|Texas Instruments Incorporated
|tmux4051, 1 Data Lane 8:1 24V Precision mux
[IBIS Ver]   4.1
[File name]   tmux4051.ibs
[Date]   05/26/22
[File Rev]   1.0
[Source]
| Texas Instruments Incorporated.
| ASC-INT-MPD
| 12500 TI Blvd
| Dallas, TX - 75243
[Notes]   Revision History:
| Rev 1.0: 05/26/22
| - Initial version of the model
| - Model generated from simulations in SPECTRE
| - C_comp although listed in numerical order of value are
|   obtained from varying PVT conditions. For PVT conditions for
|   each specific value refer the buffer description under
|   respective [Model]. IBIS model user is responsible for using
|   appropriate C_comp to simulate for Signal Integrity.
[Disclaimer]
| This model is designed as an aid for customers of Texas Instruments.
| TI and its licensors and suppliers make no warranties, either expressed
| or implied, with respect to this  model, including the warranties of
| merchantability or fitness for a particular purpose. The model is
| provided solely on an "as is" basis. The entire risk as to its quality
| and performance is with the customer.
| This model is subject to change without notice. Texas Instruments
| Incorporated is not responsible for updating this model.
[Copyright]
(C) Copyright 2022 Texas Instruments Incorporated.All rights reserved.
|  Component TMUX4051PW 16-pin - PW package
|  Part # TMUX4051PW
[Component]   TMUX4051PW
[Manufacturer]  TI
[Package]
|   typ   min   max
R_pkg   0.0668   NA   NA
L_pkg   2.1992nH   NA   NA
C_pkg   0.2884pF   NA   NA
[Pin]   signal_name   model_name
   1   S4   sterm
   2   S6   sterm
   3   D   dterm
   4   S7   sterm
   5   S5   sterm
   6   ENZ   inbuf_n
   7   VEE   power
   8   GND   gnd
   9   A2   inbuf
   10   A1   inbuf
   11   A0   inbuf
   12   S3   sterm
   13   S0   sterm
   14   S1   sterm
   15   S2   sterm
   16   VDD   power
[Series Switch Groups]
On 1 /
On 2 /
On 3 /
On 4 /
On 5 /
On 6 /
On 7 /
On 8 /
Off 1 2 3 4 5 6 7 8 /
[Series Pin Mapping]  pin_2 model_name function_table_group
|  13   3   switch_dual_5   1
|  14   3   switch_dual_5   1
|  15   3   switch_dual_5   1
|  12   3   switch_dual_5   1
|   1   3   switch_dual_5   1
|   5   3   switch_dual_5   1
|   2   3   switch_dual_5   1
|   4   3   switch_dual_5   1
|  13   3   switch_dual_12   1
|  14   3   switch_dual_12   1
|  15   3   switch_dual_12   1
|  12   3   switch_dual_12   1
|   1   3   switch_dual_12   1
|   5   3   switch_dual_12   1
|   2   3   switch_dual_12   1
|   4   3   switch_dual_12   1
|  13   3   switch_24   1
|  14   3   switch_24   1
|  15   3   switch_24   1
|  12   3   switch_24   1
|   1   3   switch_24   1
|   5   3   switch_24   1
|   2   3   switch_24   1
|   4   3   switch_24   1
|  13   3   switch_10   1
|  14   3   switch_10   1
|  15   3   switch_10   1
|  12   3   switch_10   1
|   1   3   switch_10   1
|   5   3   switch_10   1
|   2   3   switch_10   1
|   4   3   switch_10   1
  13   3   switch_5   1
  14   3   switch_5   1
  15   3   switch_5   1
  12   3   switch_5   1
   1   3   switch_5   1
   5   3   switch_5   1
   2   3   switch_5   1
   4   3   switch_5   1
|  Component TMUX4051DYY 16-pin - DYY package
|  Part # TMUX4051DYY
[Component]   TMUX4051DYY
[Manufacturer]  TI
[Package]
|   typ   min   max
R_pkg   0.0668   NA   NA
L_pkg   2.1992nH   NA   NA
C_pkg   0.2884pF   NA   NA
[Pin]   signal_name   model_name
   1   S4   sterm
   2   S6   sterm
   3   D   dterm
   4   S7   sterm
   5   S5   sterm
   6   ENZ   inbuf_n
   7   VEE   power
   8   GND   gnd
   9   A2   inbuf
   10   A1   inbuf
   11   A0   inbuf
   12   S3   sterm
   13   S0   sterm
   14   S1   sterm
   15   S2   sterm
   16   VDD   power
[Series Switch Groups]
On 1 /
On 2 /
On 3 /
On 4 /
On 5 /
On 6 /
On 7 /
On 8 /
Off 1 2 3 4 5 6 7 8 /
[Series Pin Mapping]  pin_2 model_name function_table_group
|  13   3   switch_dual_5   1
|  14   3   switch_dual_5   1
|  15   3   switch_dual_5   1
|  12   3   switch_dual_5   1
|   1   3   switch_dual_5   1
|   5   3   switch_dual_5   1
|   2   3   switch_dual_5   1
|   4   3   switch_dual_5   1
|  13   3   switch_dual_12   1
|  14   3   switch_dual_12   1
|  15   3   switch_dual_12   1
|  12   3   switch_dual_12   1
|   1   3   switch_dual_12   1
|   5   3   switch_dual_12   1
|   2   3   switch_dual_12   1
|   4   3   switch_dual_12   1
|  13   3   switch_24   1
|  14   3   switch_24   1
|  15   3   switch_24   1
|  12   3   switch_24   1
|   1   3   switch_24   1
|   5   3   switch_24   1
|   2   3   switch_24   1
|   4   3   switch_24   1
  13   3   switch_10   1
  14   3   switch_10   1
  15   3   switch_10   1
  12   3   switch_10   1
   1   3   switch_10   1
   5   3   switch_10   1
   2   3   switch_10   1
   4   3   switch_10   1
|  13   3   switch_5   1
|  14   3   switch_5   1
|  15   3   switch_5   1
|  12   3   switch_5   1
|   1   3   switch_5   1
|   5   3   switch_5   1
|   2   3   switch_5   1
|   4   3   switch_5   1
|  Component TMUX4051BQB 16-pin - BQB package
|  Part # TMUX4051BQB
[Component]   TMUX4051BQB
[Manufacturer]  TI
[Package]
|   typ   min   max
R_pkg   0.0668   NA   NA
L_pkg   2.1992nH   NA   NA
C_pkg   0.2884pF   NA   NA
[Pin]   signal_name   model_name
   1   S4   sterm
   2   S6   sterm
   3   D   dterm
   4   S7   sterm
   5   S5   sterm
   6   ENZ   inbuf_n
   7   VEE   power
   8   GND   gnd
   9   A2   inbuf
   10   A1   inbuf
   11   A0   inbuf
   12   S3   sterm
   13   S0   sterm
   14   S1   sterm
   15   S2   sterm
   16   VDD   power
[Series Switch Groups]
On 1 /
On 2 /
On 3 /
On 4 /
On 5 /
On 6 /
On 7 /
On 8 /
Off 1 2 3 4 5 6 7 8 /
[Series Pin Mapping]  pin_2 model_name function_table_group
|  13   3   switch_dual_5   1
|  14   3   switch_dual_5   1
|  15   3   switch_dual_5   1
|  12   3   switch_dual_5   1
|   1   3   switch_dual_5   1
|   5   3   switch_dual_5   1
|   2   3   switch_dual_5   1
|   4   3   switch_dual_5   1
|  13   3   switch_dual_12   1
|  14   3   switch_dual_12   1
|  15   3   switch_dual_12   1
|  12   3   switch_dual_12   1
|   1   3   switch_dual_12   1
|   5   3   switch_dual_12   1
|   2   3   switch_dual_12   1
|   4   3   switch_dual_12   1
  13   3   switch_24   1
  14   3   switch_24   1
  15   3   switch_24   1
  12   3   switch_24   1
   1   3   switch_24   1
   5   3   switch_24   1
   2   3   switch_24   1
   4   3   switch_24   1
|  13   3   switch_10   1
|  14   3   switch_10   1
|  15   3   switch_10   1
|  12   3   switch_10   1
|   1   3   switch_10   1
|   5   3   switch_10   1
|   2   3   switch_10   1
|   4   3   switch_10   1
|  13   3   switch_5   1
|  14   3   switch_5   1
|  15   3   switch_5   1
|  12   3   switch_5   1
|   1   3   switch_5   1
|   5   3   switch_5   1
|   2   3   switch_5   1
|   4   3   switch_5   1
[Model Selector] dterm
dterm_dual_5 Use for operation at +/-5V
dterm_dual_12 Use for operation at +/-12V
dterm_24 Use for operation at 24V
dterm_10 Use for operation at 10V
dterm_5 Use for operation at 5V
[Model Selector] sterm
sterm_dual_5 Use for operation at +/-5V
sterm_dual_12 Use for operation at +/-12V
sterm_24 Use for operation at 24V
sterm_10 Use for operation at 10V
sterm_5 Use for operation at 5V
[Model Selector] inbuf_n
inbuf_n_dual_5 Use for operation at +/-5V
inbuf_n_dual_12 Use for operation at +/-12V
inbuf_n_24 Use for operation at 24V
inbuf_n_10 Use for operation at 10V
inbuf_n_5 Use for operation at 5V
[Model Selector] inbuf
inbuf_dual_5 Use for operation at +/-5V
inbuf_dual_12 Use for operation at +/-12V
inbuf_24 Use for operation at 24V
inbuf_10 Use for operation at 10V
inbuf_5 Use for operation at 5V
| switch_dual_5
[Model]   switch_dual_5
Model_type   Series_switch
|   typ   min   max
C_comp   4.014581e-12   NA   NA
[Voltage Range]   5   NA   NA
[Power Clamp Reference]   5   NA   NA
[Temperature Range]   27   NA   NA
[On]
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[Off]
|   typ   min   max
[R Series]   500G   NA   NA
| switch_dual_12
[Model]   switch_dual_12
Model_type   Series_switch
|   typ   min   max
C_comp   2.533030e-12   NA   NA
[Voltage Range]   12   NA   NA
[Power Clamp Reference]   12   NA   NA
[Temperature Range]   27   NA   NA
[On]
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[Off]
|   typ   min   max
[R Series]   500G   NA   NA
| switch_24
[Model]   switch_24
Model_type   Series_switch
|   typ   min   max
C_comp   2.533030e-12   NA   NA
[Voltage Range]   24   NA   NA
[Power Clamp Reference]   24   NA   NA
[Temperature Range]   27   NA   NA
[On]
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[Off]
|   typ   min   max
[R Series]   500G   NA   NA
| switch_10
[Model]   switch_10
Model_type   Series_switch
|   typ   min   max
C_comp   4.014581e-12   NA   NA
[Voltage Range]   10   NA   NA
[Power Clamp Reference]   10   NA   NA
[Temperature Range]   27   NA   NA
[On]
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[Off]
|   typ   min   max
[R Series]   500G   NA   NA
| switch_5
[Model]   switch_5
Model_type   Series_switch
|   typ   min   max
C_comp   4.014581e-12   NA   NA
[Voltage Range]   5   NA   NA
[Power Clamp Reference]   5   NA   NA
[Temperature Range]   27   NA   NA
[On]
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[Off]
|   typ   min   max
[R Series]   500G   NA   NA
| Models and submodels in the file (25): dterm_dual_5 (Terminator), dterm_dual_12 (Terminator), dterm_24 (Terminator), dterm_10 (Terminator), dterm_5 (Terminator), switch_dual_5 (Series_switch), switch_dual_12 (Series_switch), switch_24 (Series_switch), switch_10 (Series_switch), switch_5 (Series_switch), sterm_dual_5 (Terminator), sterm_dual_12 (Terminator), sterm_24 (Terminator), sterm_10 (Terminator), sterm_5 (Terminator), inbuf_dual_5 (Input), inbuf_dual_12 (Input), inbuf_24 (Input), inbuf_10 (Input), inbuf_5 (Input), inbuf_n_dual_5 (Input), inbuf_n_dual_12 (Input), inbuf_n_24 (Input), inbuf_n_10 (Input), inbuf_n_5 (Input)
